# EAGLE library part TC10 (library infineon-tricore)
+ Obsolete + TC10 GP TriCore 32bit Microcontroller+ DSP Source: http://www.infineon.com ..
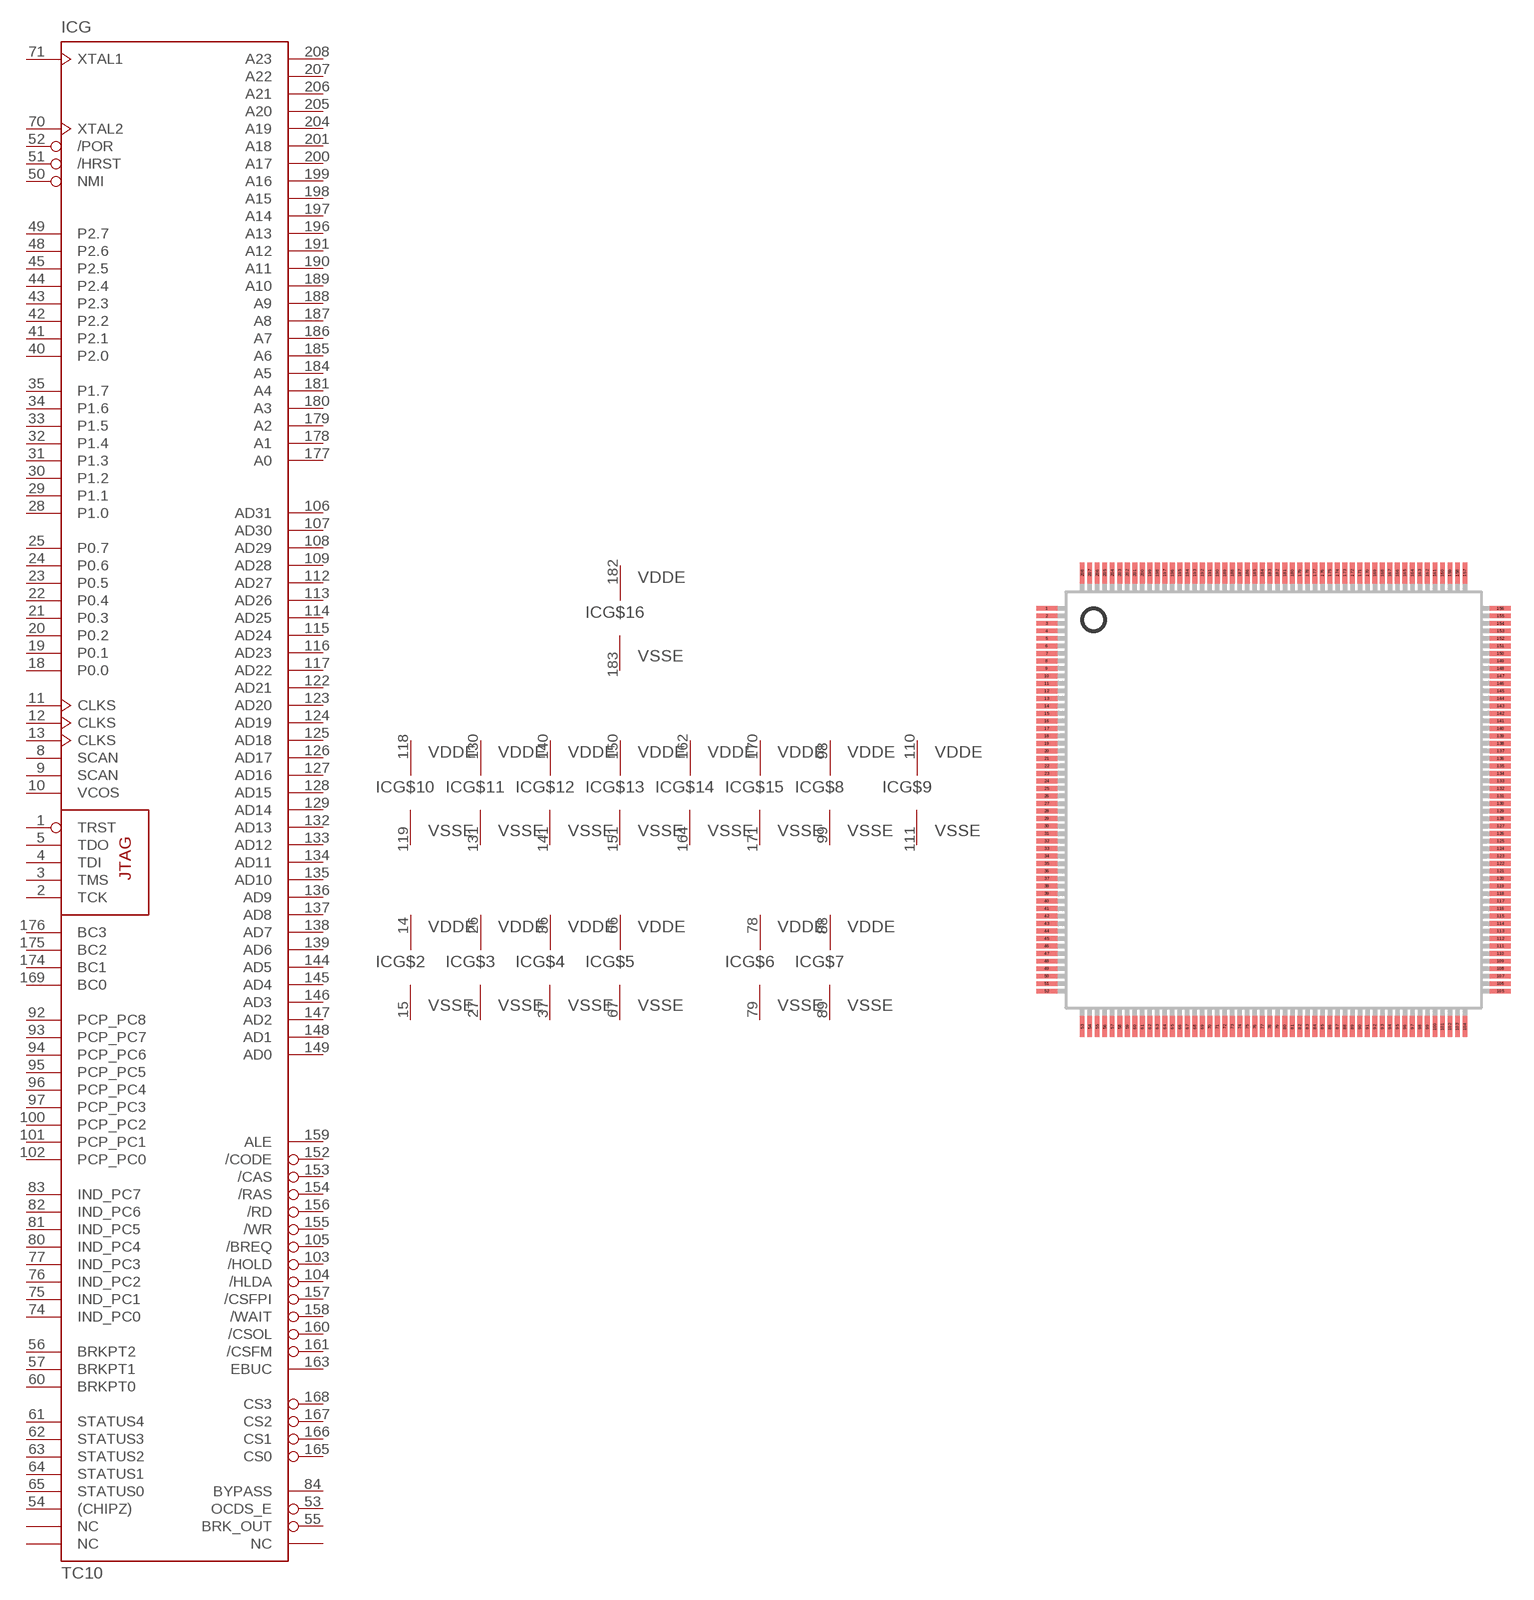
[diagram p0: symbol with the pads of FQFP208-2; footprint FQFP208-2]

Designator prefix IC; gates G=TC10 G$2=VSSE_VDD G$3=VSSE_VDD G$4=VSSE_VDD G$5=VSSE_VDD G$6=VSSE_VDD G$7=VSSE_VDD G$8=VSSE_VDD G$9=VSSE_VDD G$10=VSSE_VDD G$11=VSSE_VDD G$12=VSSE_VDD G$13=VSSE_VDD G$14=VSSE_VDD G$15=VSSE_VDD G$16=VSSE_VDD G$17=VSSE_VDD G$18=VSSE_VDD G$19=VSSE_VDD G$20=VSSE_VDD G$21=VSS_VDD G$22=VSS_VDD G$23=VSS_VDD G$24=VSS_VDD G$25=VSS_VDD G$26=VSS_VDD G$27=VSS_VDD G$28=VSSP_VDD G$1=VSSE_VDD G$29=VSS_VDD

## TC10 (OC_FARNELL: unknown; OC_NEWARK: unknown)  [FQFP208-2]
1  G:TRST  in
2  G:TCK  in
3  G:TMS  in
4  G:TDI  in
5  G:TDO  in
6  G$1:VDDE  pwr
7  G$1:VSSE  pwr
8  G:SCAN  in
9  G:SCAN  in
10  G:VCOS  in
11  G:CLKS  in
12  G:CLKS  in
13  G:CLKS  in
14  G$2:VDDE  pwr
15  G$2:VSSE  pwr
16  G$21:VSS  pwr
17  G$21:VDD  pwr
18  G:P0.0
19  G:P0.1
20  G:P0.2
21  G:P0.3
22  G:P0.4
23  G:P0.5
24  G:P0.6
25  G:P0.7
26  G$3:VDDE  pwr
27  G$3:VSSE  pwr
28  G:P1.0
29  G:P1.1
30  G:P1.2
31  G:P1.3
32  G:P1.4
33  G:P1.5
34  G:P1.6
35  G:P1.7
36  G$4:VDDE  pwr
37  G$4:VSSE  pwr
38  G$22:VSS  pwr
39  G$22:VDD  pwr
40  G:P2.0
41  G:P2.1
42  G:P2.2
43  G:P2.3
44  G:P2.4
45  G:P2.5
46  G$18:VDDE  pwr
47  G$18:VSSE  pwr
48  G:P2.6
49  G:P2.7
50  G:NMI  in
51  G:/HRST  in
52  G:/POR  in
53  G:OCDS_E  out
54  G:(CHIPZ)
55  G:BRK_OUT  out
56  G:BRKPT2
57  G:BRKPT1
58  G$19:VDDE  pwr
59  G$19:VSSE  pwr
60  G:BRKPT0
61  G:STATUS4
62  G:STATUS3
63  G:STATUS2
64  G:STATUS1
65  G:STATUS0
66  G$5:VDDE  pwr
67  G$5:VSSE  pwr
68  G$23:VSS  pwr
69  G$23:VDD  pwr
70  G:XTAL2  out
71  G:XTAL1  in
72  G$28:VSSP  pwr
73  G$28:VDDP  pwr
74  G:IND_PC0
75  G:IND_PC1
76  G:IND_PC2
77  G:IND_PC3
78  G$6:VDDE  pwr
79  G$6:VSSE  pwr
80  G:IND_PC4
81  G:IND_PC5
82  G:IND_PC6
83  G:IND_PC7
84  G:BYPASS
85  G:NC  nc
86  G:NC  nc
87  G:NC  nc
88  G$7:VDDE  pwr
89  G$7:VSSE  pwr
90  G$24:VSS  pwr
91  G$24:VDD  pwr
92  G:PCP_PC8
93  G:PCP_PC7
94  G:PCP_PC6
95  G:PCP_PC5
96  G:PCP_PC4
97  G:PCP_PC3
98  G$8:VDDE  pwr
99  G$8:VSSE  pwr
100  G:PCP_PC2
101  G:PCP_PC1
102  G:PCP_PC0
103  G:/HOLD  out
104  G:/HLDA  out
105  G:/BREQ  out
106  G:AD31
107  G:AD30
108  G:AD29
109  G:AD28
110  G$9:VDDE  pwr
111  G$9:VSSE  pwr
112  G:AD27
113  G:AD26
114  G:AD25
115  G:AD24
116  G:AD23
117  G:AD22
118  G$10:VDDE  pwr
119  G$10:VSSE  pwr
120  G$25:VSS  pwr
121  G$25:VDD  pwr
122  G:AD21
123  G:AD20
124  G:AD19
125  G:AD18
126  G:AD17
127  G:AD16
128  G:AD15
129  G:AD14
130  G$11:VDDE  pwr
131  G$11:VSSE  pwr
132  G:AD13
133  G:AD12
134  G:AD11
135  G:AD10
136  G:AD9
137  G:AD8
138  G:AD7
139  G:AD6
140  G$12:VDDE  pwr
141  G$12:VSSE  pwr
142  G$26:VSS  pwr
143  G$26:VDD  pwr
144  G:AD5
145  G:AD4
146  G:AD3
147  G:AD2
148  G:AD1
149  G:AD0
150  G$13:VDDE  pwr
151  G$13:VSSE  pwr
152  G:/CODE  out
153  G:/CAS  out
154  G:/RAS  out
155  G:/WR  out
156  G:/RD  out
157  G:/CSFPI  out
158  G:/WAIT  out
159  G:ALE  out
160  G:/CSOL  out
161  G:/CSFM  out
162  G$14:VDDE  pwr
163  G:EBUC  out
164  G$14:VSSE  pwr
165  G:CS0  out
166  G:CS1  out
167  G:CS2  out
168  G:CS3  out
169  G:BC0
170  G$15:VDDE  pwr
171  G$15:VSSE  pwr
172  G$27:VSS  pwr
173  G$27:VDD  pwr
174  G:BC1
175  G:BC2
176  G:BC3
177  G:A0  out
178  G:A1  out
179  G:A2  out
180  G:A3  out
181  G:A4  out
182  G$16:VDDE  pwr
183  G$16:VSSE  pwr
184  G:A5  out
185  G:A6  out
186  G:A7  out
187  G:A8  out
188  G:A9  out
189  G:A10  out
190  G:A11  out
191  G:A12  out
192  G$20:VDDE  pwr
193  G$20:VSSE  pwr
194  G$29:VSS  pwr
195  G$29:VDD  pwr
196  G:A13  out
197  G:A14  out
198  G:A15  out
199  G:A16  out
200  G:A17  out
201  G:A18  out
202  G$17:VDDE  pwr
203  G$17:VSSE  pwr
204  G:A19  out
205  G:A20  out
206  G:A21  out
207  G:A22  out
208  G:A23  out

## Footprint FQFP208-2 (pad centres in mm)
P-FQFP-208-2, -4, -7 Plastic Fine Pitch Quad Flat Package Source: http://www.infineon.com
smd 1.4 x 0.31: 1 -15.125,12.75; 2 -15.125,12.25; 3 -15.125,11.75; 4 -15.125,11.25; 5 -15.125,10.75; 6 -15.125,10.25; 7 -15.125,9.75; 8 -15.125,9.25; 9 -15.125,8.75; 10 -15.125,8.25; 11 -15.125,7.75; 12 -15.125,7.25; 13 -15.125,6.75; 14 -15.125,6.25; 15 -15.125,5.75; 16 -15.125,5.25; 17 -15.125,4.75; 18 -15.125,4.25; 19 -15.125,3.75; 20 -15.125,3.25; 21 -15.125,2.75; 22 -15.125,2.25; 23 -15.125,1.75; 24 -15.125,1.25; 25 -15.125,0.75; 26 -15.125,0.25; 27 -15.125,-0.25; 28 -15.125,-0.75; 29 -15.125,-1.25; 30 -15.125,-1.75; 31 -15.125,-2.25; 32 -15.125,-2.75; 33 -15.125,-3.25; 34 -15.125,-3.75; 35 -15.125,-4.25; 36 -15.125,-4.75; 37 -15.125,-5.25; 38 -15.125,-5.75; 39 -15.125,-6.25; 40 -15.125,-6.75; 41 -15.125,-7.25; 42 -15.125,-7.75; 43 -15.125,-8.25; 44 -15.125,-8.75; 45 -15.125,-9.25; 46 -15.125,-9.75; 47 -15.125,-10.25; 48 -15.125,-10.75; 49 -15.125,-11.25; 50 -15.125,-11.75; 51 -15.125,-12.25; 52 -15.125,-12.75; 105 15.125,-12.75; 106 15.125,-12.25; 107 15.125,-11.75; 108 15.125,-11.25; 109 15.125,-10.75; 110 15.125,-10.25; 111 15.125,-9.75; 112 15.125,-9.25; 113 15.125,-8.75; 114 15.125,-8.25; 115 15.125,-7.75; 116 15.125,-7.25; 117 15.125,-6.75; 118 15.125,-6.25; 119 15.125,-5.75; 120 15.125,-5.25; 121 15.125,-4.75; 122 15.125,-4.25; 123 15.125,-3.75; 124 15.125,-3.25; 125 15.125,-2.75; 126 15.125,-2.25; 127 15.125,-1.75; 128 15.125,-1.25; 129 15.125,-0.75; 130 15.125,-0.25; 131 15.125,0.25; 132 15.125,0.75; 133 15.125,1.25; 134 15.125,1.75; 135 15.125,2.25; 136 15.125,2.75; 137 15.125,3.25; 138 15.125,3.75; 139 15.125,4.25; 140 15.125,4.75; 141 15.125,5.25; 142 15.125,5.75; 143 15.125,6.25; 144 15.125,6.75; 145 15.125,7.25; 146 15.125,7.75; 147 15.125,8.25; 148 15.125,8.75; 149 15.125,9.25; 150 15.125,9.75; 151 15.125,10.25; 152 15.125,10.75; 153 15.125,11.25; 154 15.125,11.75; 155 15.125,12.25; 156 15.125,12.75
smd 0.31 x 1.4: 53 -12.75,-15.125; 54 -12.25,-15.125; 55 -11.75,-15.125; 56 -11.25,-15.125; 57 -10.75,-15.125; 58 -10.25,-15.125; 59 -9.75,-15.125; 60 -9.25,-15.125; 61 -8.75,-15.125; 62 -8.25,-15.125; 63 -7.75,-15.125; 64 -7.25,-15.125; 65 -6.75,-15.125; 66 -6.25,-15.125; 67 -5.75,-15.125; 68 -5.25,-15.125; 69 -4.75,-15.125; 70 -4.25,-15.125; 71 -3.75,-15.125; 72 -3.25,-15.125; 73 -2.75,-15.125; 74 -2.25,-15.125; 75 -1.75,-15.125; 76 -1.25,-15.125; 77 -0.75,-15.125; 78 -0.25,-15.125; 79 0.25,-15.125; 80 0.75,-15.125; 81 1.25,-15.125; 82 1.75,-15.125; 83 2.25,-15.125; 84 2.75,-15.125; 85 3.25,-15.125; 86 3.75,-15.125; 87 4.25,-15.125; 88 4.75,-15.125; 89 5.25,-15.125; 90 5.75,-15.125; 91 6.25,-15.125; 92 6.75,-15.125; 93 7.25,-15.125; 94 7.75,-15.125; 95 8.25,-15.125; 96 8.75,-15.125; 97 9.25,-15.125; 98 9.75,-15.125; 99 10.25,-15.125; 100 10.75,-15.125; 101 11.25,-15.125; 102 11.75,-15.125; 103 12.25,-15.125; 104 12.75,-15.125; 157 12.75,15.125; 158 12.25,15.125; 159 11.75,15.125; 160 11.25,15.125; 161 10.75,15.125; 162 10.25,15.125; 163 9.75,15.125; 164 9.25,15.125; 165 8.75,15.125; 166 8.25,15.125; 167 7.75,15.125; 168 7.25,15.125; 169 6.75,15.125; 170 6.25,15.125; 171 5.75,15.125; 172 5.25,15.125; 173 4.75,15.125; 174 4.25,15.125; 175 3.75,15.125; 176 3.25,15.125; 177 2.75,15.125; 178 2.25,15.125; 179 1.75,15.125; 180 1.25,15.125; 181 0.75,15.125; 182 0.25,15.125; 183 -0.25,15.125; 184 -0.75,15.125; 185 -1.25,15.125; 186 -1.75,15.125; 187 -2.25,15.125; 188 -2.75,15.125; 189 -3.25,15.125; 190 -3.75,15.125; 191 -4.25,15.125; 192 -4.75,15.125; 193 -5.25,15.125; 194 -5.75,15.125; 195 -6.25,15.125; 196 -6.75,15.125; 197 -7.25,15.125; 198 -7.75,15.125; 199 -8.25,15.125; 200 -8.75,15.125; 201 -9.25,15.125; 202 -9.75,15.125; 203 -10.25,15.125; 204 -10.75,15.125; 205 -11.25,15.125; 206 -11.75,15.125; 207 -12.25,15.125; 208 -12.75,15.125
